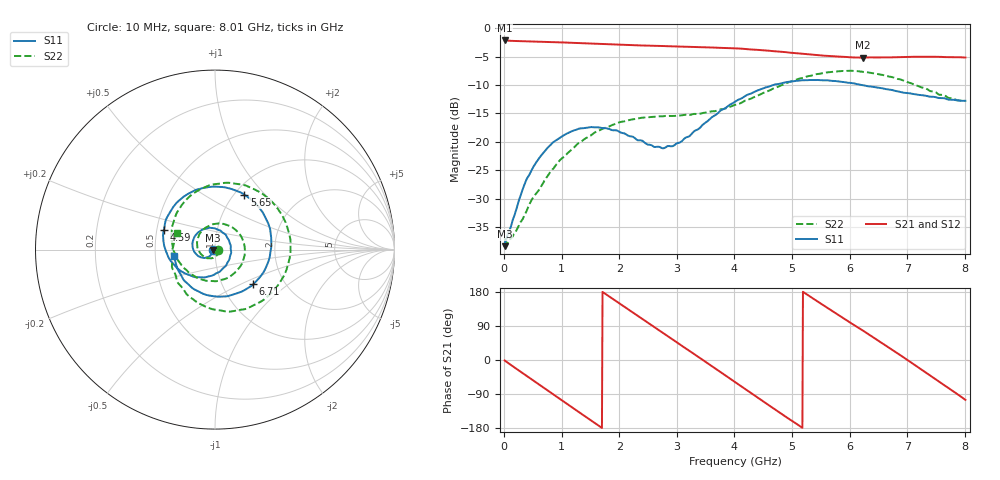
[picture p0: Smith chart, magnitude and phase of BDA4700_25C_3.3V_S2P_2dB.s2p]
!Agilent Technologies,E5071B,MY42404982,A.09.10
!Date: Mon Oct 20 18:03:49 2025
!Data & Calibration Information:
!Freq	S11:SOLT2(ON)	S21:SOLT2(ON)	S12:SOLT2(ON)	S22:SOLT2(ON)
# Hz S RI R 50
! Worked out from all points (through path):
!   801 points, 10 MHz to 8.01 GHz, reference 50 ohm
!   highest |S21| = -2.11 dB at 10 MHz (marker M1); lowest = -5.1 dB at 6.23 GHz (marker M2)
!   group delay of S21, straight-line fit = 285 ps
!   lowest |S11| = -38.4 dB at 10 MHz (marker M3), VSWR 1.02, Z = 48.8 - j0.183 ohm
!   |S11| at or under -10 dB: start of sweep to 4.668 GHz; 6.226 GHz to end of sweep
!   |S22| runs from -37.9 to -7.5 dB; largest |S21 - S12| = 0.009
!   S11 on the Smith chart (normalised r, x): 10 MHz: 0.98, -0.00; 4.59 GHz: 0.54, +0.13; 5.65 GHz: 1.11, +0.77; 6.71 GHz: 1.40, -0.59; 8.01 GHz: 0.63, -0.05
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1e7  -0.0119 -0.00187  0.7837 -0.0167  0.7835 -0.0172  0.014 -0.00151
3.7e8  -0.0272 -0.0345  0.5938 -0.4919  0.5932 -0.4917  0.0151 -0.0177
7.1e8  -0.0697 -0.0453  0.1904 -0.7374  0.19 -0.7377  -0.00872 -0.0452
1.02e9  -0.1115 -0.0175  -0.234 -0.7152  -0.2342 -0.7152  -0.0595 -0.0411
1.35e9  -0.1244 0.0423  -0.5905 -0.4494  -0.5908 -0.45  -0.0991 0.0217
1.64e9  -0.0949 0.0949  -0.7269 -0.0892  -0.7273 -0.0899  -0.0779 0.098
1.93e9  -0.0377 0.1208  -0.6638 0.2839  -0.6644 0.2838  0.00315 0.1438
2.32e9  0.0442 0.0934  -0.319 0.6346  -0.3189 0.6349  0.1271 0.0983
2.68e9  0.0871 0.0247  0.1267 0.6903  0.1255 0.6902  0.1653 -0.0291
3.37e9  0.0142 -0.1283  0.6782 0.1007  0.6791 0.101  -0.016 -0.175
3.67e9  -0.0762 -0.1543  0.6255 -0.2606  0.6253 -0.2623  -0.116 -0.1468
4.01e9  -0.1934 -0.117  0.3522 -0.5666  0.3532 -0.5656  -0.2008 -0.0671
4.59e9  -0.2853 0.1114  -0.3054 -0.559  -0.3041 -0.5603  -0.2273 0.1648
4.98e9  -0.1882 0.2836  -0.5688 -0.2221  -0.5698 -0.2242  -0.1008 0.3254
5.35e9  0.00143 0.3507  -0.5647 0.1638  -0.5655 0.1608  0.1204 0.3663
5.65e9  0.1642 0.3055  -0.3981 0.4095  -0.3975 0.4098  0.3002 0.2818
6.23e9  0.3143 0.0327  0.1185 0.5402  0.1264 0.539  0.4037 -0.0935
6.68e9  0.2237 -0.1832  0.4682 0.3001  0.4701 0.2995  0.2078 -0.3142
6.71e9  0.2133 -0.1936  0.4832 0.2755  0.4852 0.2744  0.1895 -0.3232
7.27e9  -0.0433 -0.2537  0.4999 -0.2608  0.4991 -0.2611  -0.1345 -0.2687
7.65e9  -0.178 -0.1643  0.2174 -0.5157  0.2163 -0.5164  -0.24 -0.0916
8.01e9  -0.2273 -0.0357  -0.1448 -0.5351  -0.1428 -0.5358  -0.2099 0.093
